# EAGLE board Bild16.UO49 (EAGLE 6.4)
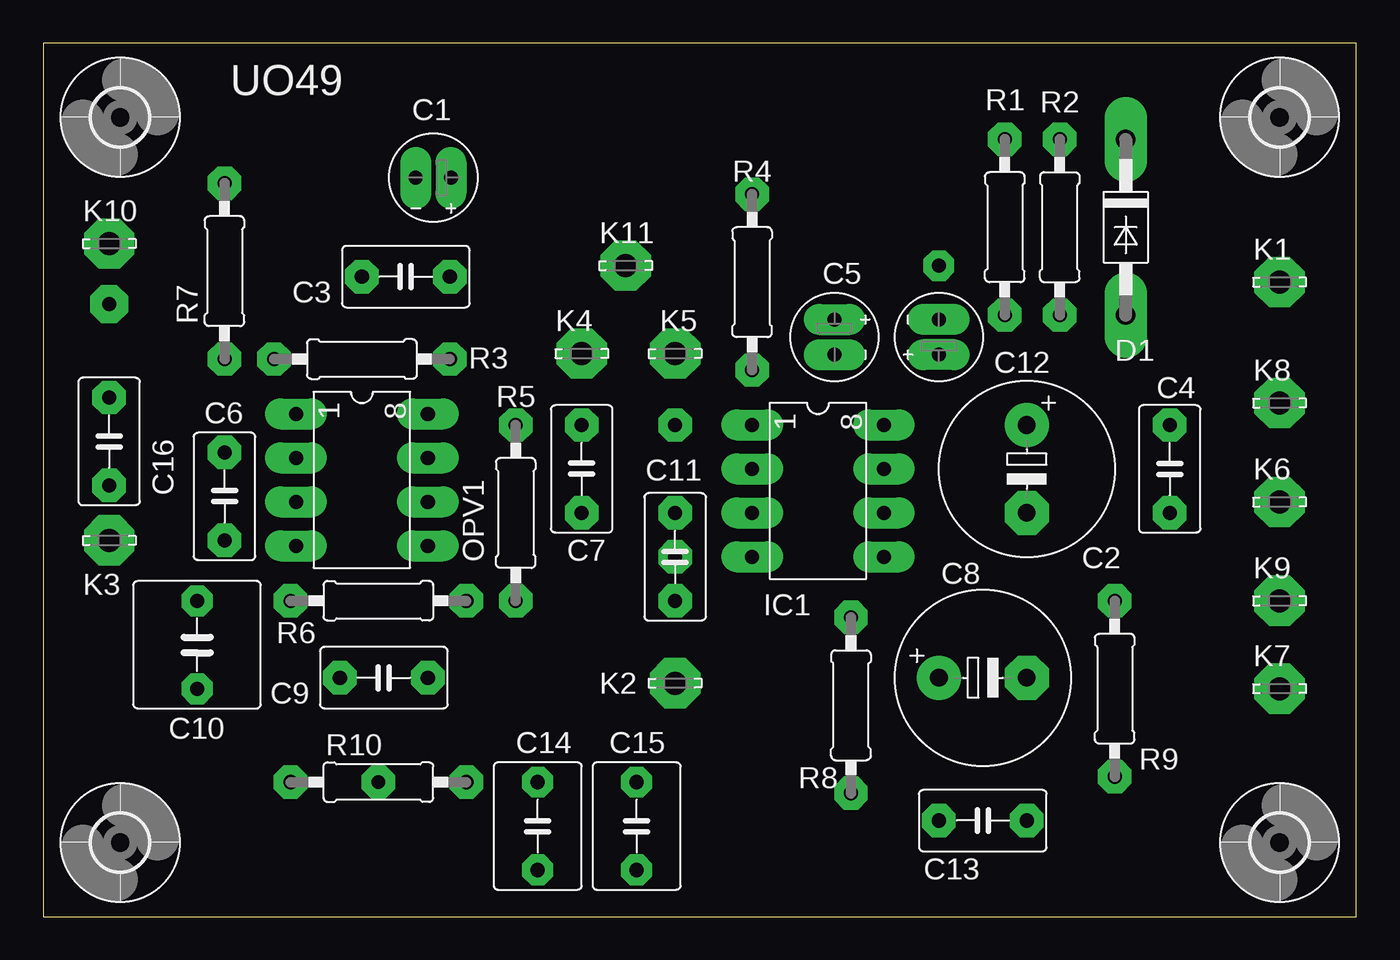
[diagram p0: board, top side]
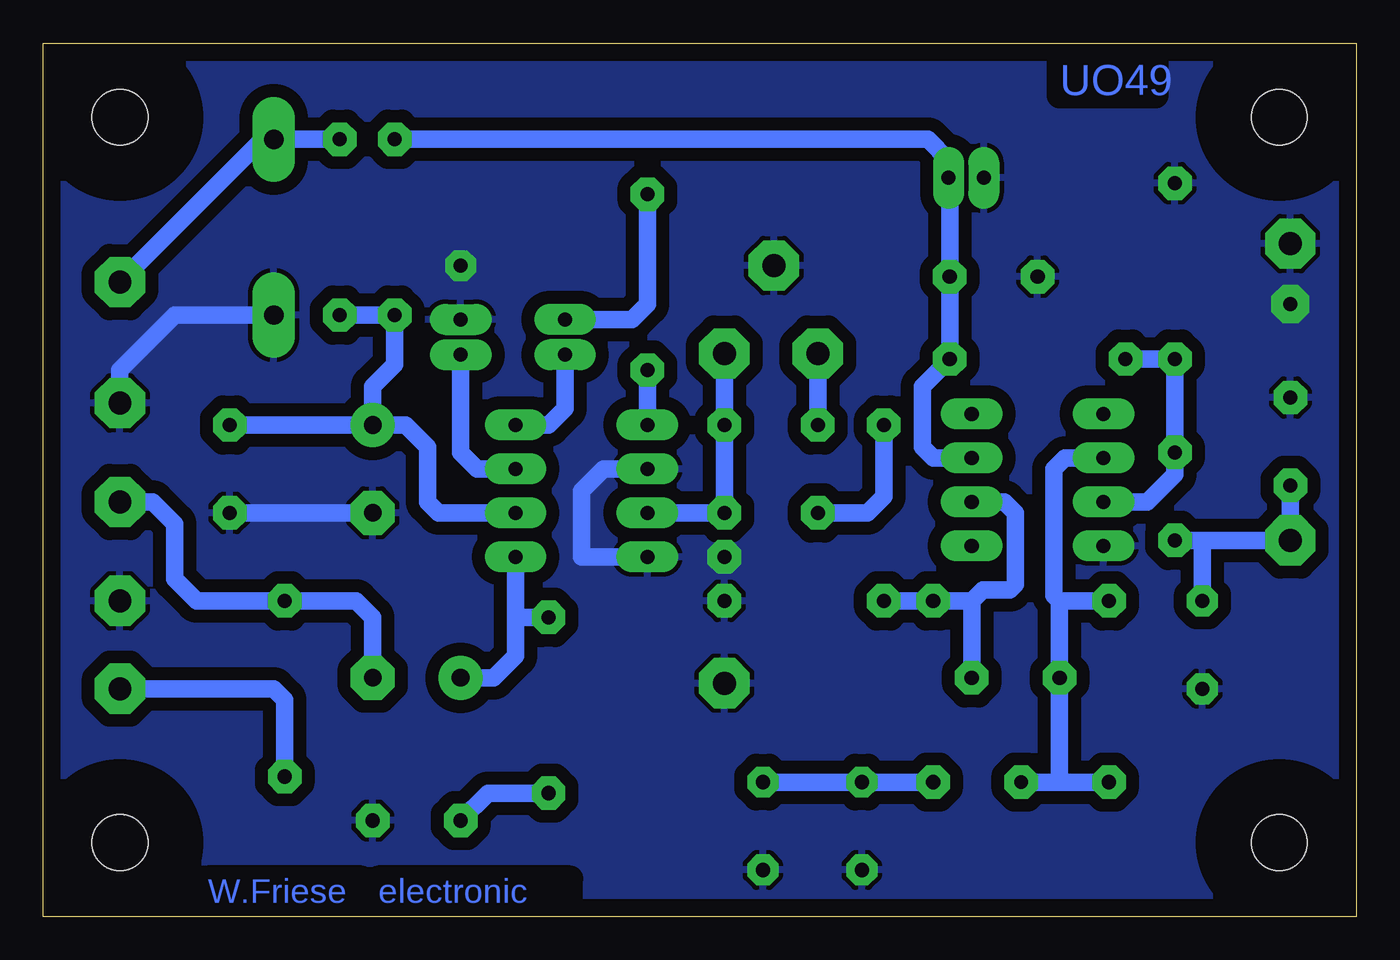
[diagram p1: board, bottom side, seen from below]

Size 75.86 x 50.47 mm. Coordinates in mm from the lower left corner, seen from the top.
Outline: 0,0 75.86,0 75.86,50.47 0,50.47 0,0
Copper layers (1*16): Top 0.035mm / dielectric 1.5mm / Bottom 0.035mm
Design rules "default *": minimum track width 10mil, minimum drill 24mil, track to track 8mil, track to pad 8mil, pad to pad 8mil, via to via 8mil, smd to smd 8mil, copper to edge 40mil, drill to drill 8mil, minimum pad ring 10mil, minimum via ring 8mil, stop-mask expansion 0mil, vias tented up to drill 0mil, thermal gap 10mil

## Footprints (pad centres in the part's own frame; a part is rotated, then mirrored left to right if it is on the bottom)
E2-5 = drill 0.813 pad 1.27 long: + -1.016,0; - 1.016,0
E5-10,5 = drill 1.016 pad 2.54: + -2.54,0 | drill 1.016 pad 2.54 octagon: - 2.54,0
C050-035X075 = drill 0.813 pad 1.93 octagon: 1 -2.54,0; 2 2.54,0
C050-075X075 = drill 0.813 octagon: 1 -2.54,0; 2 2.54,0
C050-050X075 = drill 0.813 octagon: 1 -2.54,0; 2 2.54,0
DO41-10 = drill 1.118 long: A 5.08,0; K -5.08,0
3,2 = hole 3.2: 0,0
DIL08 = drill 0.813 long: 1 -3.81,-3.81; 2 -1.27,-3.81; 3 1.27,-3.81; 4 3.81,-3.81; 5 3.81,3.81; 6 1.27,3.81; 7 -1.27,3.81; 8 -3.81,3.81
LSP13 = drill 1.321 pad 2.159 octagon: MP 0,0
DIL08@1 = drill 0.813 long: 1 -3.81,-3.81; 2 -1.27,-3.81; 3 1.27,-3.81; 4 3.81,-3.81; 5 3.81,3.81; 6 1.27,3.81; 7 -1.27,3.81; 8 -3.81,3.81
0207/10E = drill 0.813 pad 1.93 octagon: 1 -4.445,0; 2 5.715,0

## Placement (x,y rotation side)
C1  [E2-5]  22.54,42.7 180 top
C2  [E5-10,5]  56.83,25.87 270 top
C3  [C050-035X075]  20.95,36.98 180 top
C4  [C050-035X075]  65.08,25.87 270 top
C5  [E2-5]  45.71,33.49 270 top
C6  [C050-035X075]  10.47,24.28 90 top
C7  [C050-035X075]  31.11,25.87 90 top
C8  [E5-10,5]  54.29,13.81 0 top
C9  [C050-035X075]  19.68,13.81 180 top
C10  [C050-075X075]  8.88,15.71 90 top
C11  [C050-035X075]  36.51,20.79 270 top
C12  [E2-5]  51.75,33.49 90 top
C13  [C050-035X075]  54.29,5.55 0 top
C14  [C050-050X075]  28.57,5.23 270 top
C15  [C050-050X075]  34.28,5.23 270 top
C16  [C050-035X075]  3.81,27.46 270 top
D1  [DO41-10]  62.54,39.84 270 top
H1  MOUNT-HOLE3.2  [3,2]  71.43,4.28 0 top
H2  MOUNT-HOLE3.2  [3,2]  71.43,46.19 0 top
H3  MOUNT-HOLE3.2  [3,2]  4.44,4.28 0 top
H4  MOUNT-HOLE3.2  [3,2]  4.44,46.19 0 top
IC1  [DIL08]  44.76,24.6 270 top
K1  LSP13  [LSP13]  71.43,36.66 0 top
K2  LSP13  [LSP13]  36.51,13.49 0 top
K3  LSP13  [LSP13]  3.81,21.74 0 top
K4  LSP13  [LSP13]  31.11,32.54 0 top
K5  LSP13  [LSP13]  36.51,32.54 0 top
K6  LSP13  [LSP13]  71.43,23.96 0 top
K7  LSP13  [LSP13]  71.43,13.17 0 top
K8  LSP13  [LSP13]  71.43,29.68 0 top
K9  LSP13  [LSP13]  71.43,18.25 0 top
K10  LSP13  [LSP13]  3.81,38.89 0 top
K11  LSP13  [LSP13]  33.65,37.62 0 top
OPV1  [DIL08@1]  18.41,25.23 270 top
R1  [0207/10E]  55.56,39.2 90 top
R2  [0207/10E]  58.73,40.48 270 top
R3  [0207/10E]  19.05,32.22 180 top
R4  [0207/10E]  40.95,36.03 90 top
R5  [0207/10E]  27.3,22.7 90 top
R6  [0207/10E]  20,18.25 180 top
R7  [0207/10E]  10.47,36.66 90 top
R8  [0207/10E]  46.67,12.85 270 top
R9  [0207/10E]  61.91,12.54 90 top
R10  [0207/10E]  18.73,7.77 0 top

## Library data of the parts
C1-C16 R1-R10 = rcl
D1 = diode
H1-H4 = holes
IC1 OPV1 = linear
K1-K11 = solpad

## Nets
GND: C1.- C2.- C3.2 C4.2 C10.1 C11.2 C12.- C13.2 C14.2 C15.2 C16.1 D1.A IC1.2 IC1.4 K2.MP K8.MP K9.MP K10.MP K11.MP OPV1.4 R7.2
N$1: D1.K K1.MP R2.1
N$2: K7.MP R9.1
N$3: C8.+ IC1.5 R8.1
N$4: C12.+ IC1.7
N$5: IC1.1 R4.1
N$6: C11.1 IC1.3 K5.MP
N$7: C2.+ C4.1 IC1.6 R1.1 R2.2
N$8: C13.1 R8.2
N$9: C8.- K6.MP R9.2
N$10: C5.+ R4.2
N$11: C5.- IC1.8
N$13: C1.+ C3.1 OPV1.7 R1.2 R3.1
N$14: C7.1 R5.2
N$15: C7.2 K4.MP
N$16: C14.1 C15.1 R10.2
N$17: C9.2 OPV1.2 R6.2 R10.1
N$19: C9.1 OPV1.6 R5.1 R6.1
N$20: C6.2 OPV1.3 R3.2 R7.1
N$22: C6.1 C10.2 C16.2 K3.MP

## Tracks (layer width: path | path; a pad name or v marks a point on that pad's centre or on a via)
GND  (via drill 0.8, 0.8 pad 1.93, 0.8 pad 2.18)
  Bottom 1.016: D1.A 68.26,34.76 71.43,31.59 K8.MP | C2.- C4.2 | IC1.2 43.49,25.87 44.76,24.6 44.76,20.79 IC1.4
  other vias: 51.75,37.62 36.51,20.79 3.81,35.4
  pour Bottom (isolate 0.75): -0.01,-0.17 75.88,-0.17 75.88,50.63 -0.01,50.63
N$1
  Bottom 1.016: R2.1 D1.K 63.18,44.92 K1.MP
N$2
  Bottom 1.016: K7.MP 62.54,13.17 61.91,12.54 R9.1
N$3
  Bottom 1.016: IC1.5 48.57,17.3 | 48.57,17.3 48.57,15.08 49.84,13.81 C8.+ | R8.1 48.57,17.3
N$4
  Bottom 1.016: IC1.7 50.79,25.87 51.75,26.82 C12.+
N$5
  Bottom 1.016: IC1.1 R4.1
N$6
  Bottom 1.016: IC1.3 C11.1 K5.MP
N$7
  Bottom 1.016: C2.+ 54.92,28.41 53.65,27.14 53.65,23.96 53.02,23.33 IC1.6 | C2.+ C4.1 | R2.2 R1.1 55.56,31.9 56.83,30.63 C2.+
N$8
  Bottom 1.016: R8.2 50.16,7.14 C13.1
N$9
  Bottom 1.016: K6.MP 69.53,23.96 68.26,22.7 68.26,19.52 66.99,18.25 R9.2 57.78,18.25 56.83,17.3 C8.-
N$10
  Bottom 1.016: C5.+ 41.84,34.51 40.95,35.4 R4.2
N$11
  Bottom 1.016: C5.- 45.71,29.36 46.67,28.41 IC1.8
N$12  (via drill 0.8 pad 1.93)
  other vias: 36.51,28.41
N$13
  Bottom 1.016: R1.2 24.76,44.92 23.55,43.71 C1.+ 23.49,42.63 C3.1 R3.1 25.08,30.63 25.08,27.14 24.44,26.51 OPV1.7
N$14
  Bottom 1.016: R5.2 27.3,24.28 28.25,23.33 C7.1
N$15
  Bottom 1.016: C7.2 K4.MP
N$16
  Bottom 1.016: R10.2 C14.1 C15.1
N$17
  Bottom 1.016: 17.14,18.25 17.46,18.57 17.46,25.87 16.82,26.51 OPV1.2 | 17.14,18.25 R6.2 | 17.14,18.25 C9.2 17.14,8.09 17.46,7.77 | 17.46,7.77 R10.1 | 19.68,7.77 17.46,7.77
N$18  (via drill 0.8 pad 1.93)
  other vias: 19.36,7.77
N$19
  Bottom 1.016: 22.22,18.25 21.59,18.89 20,18.89 19.68,19.2 19.68,23.33 20.32,23.96 OPV1.6 | 22.22,18.25 R6.1 R5.1 | C9.1 22.22,18.25
N$20
  Bottom 1.016: R3.2 R7.1 C6.2 10.47,25.55 12.06,23.96 OPV1.3
N$22
  Bottom 1.016: C6.1 9.2,21.74 | 9.2,21.74 K3.MP C16.2 | C10.2 8.88,21.43 9.2,21.74

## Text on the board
Bottom: UO49 | electronic | W.Friese
tPlace: UO49
_tNames: R1 | C1 | R2 | R4 | K10 | K11 | K1 | C3 | C5 | R7 | K4 | K5 | R3 | C12 | D1 | R5 | K8 | C6 | C4 | C16 | OPV1 | K6 | C7 | C2 | K9 | K3 | C8 | IC1 | R6 | C11 | K7 | C9 | K2 | C10 | C14 | C15 | R9 | R10 | R8 | C13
